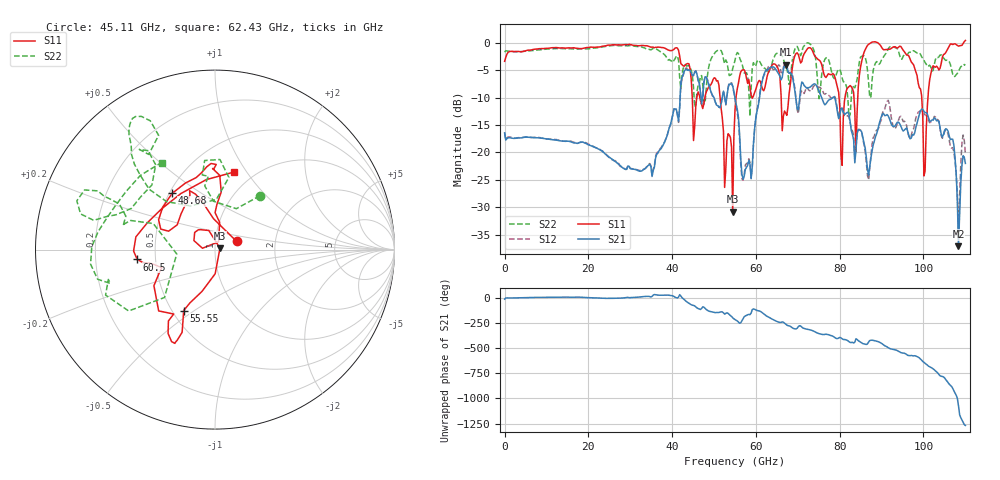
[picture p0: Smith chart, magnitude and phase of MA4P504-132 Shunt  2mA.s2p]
!Keysight Technologies,N5247B,US61255204,A.15.70.20
!Date: Friday, October 21, 2022 14:56:18
!Correction: S11(C  4-Port  )
!S31(C  4-Port  )
!S13(C  4-Port  )
!S33(C  4-Port  )
!S2P File: Measurements: S11, S31, S13, S33:
# Hz S  dB  R 50
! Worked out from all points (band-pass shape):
!   401 points, 10 MHz to 110 GHz, reference 50 ohm
!   highest |S21| = -3.99 dB at 67.1 GHz (marker M1); lowest = -37.1 dB at 108.4 GHz (marker M2)
!   |S21| within 3 dB of the highest: 42.15 GHz to 46.28 GHz (4.135 GHz wide, 9.35 % of centre); 61.5 GHz to 68.91 GHz (7.411 GHz wide, 11.4 % of centre)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
!   lowest |S11| = -30.8 dB at 54.46 GHz (marker M3), VSWR 1.06, Z = 52.8 + j0.811 ohm
!   |S11| at or under -10 dB: 51.45 GHz to 55.25 GHz (3.792 GHz wide, 7.11 % of centre); 66.02 GHz to 67.84 GHz (1.818 GHz wide, 2.72 % of centre); 79.85 GHz to 81.26 GHz (1.412 GHz wide, 1.75 % of centre)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
!   |S22| runs from -13.5 to 0.0 dB; largest |S21 - S12| = 0.24
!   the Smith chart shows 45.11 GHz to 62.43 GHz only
!   S11 on the Smith chart (normalised r, x): 45.11 GHz: 1.27, +0.12; 48.68 GHz: 0.52, +0.38; 55.55 GHz: 0.57, -0.45; 60.5 GHz: 0.39, -0.05; 62.43 GHz: 0.81, +0.88
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1e7  -3.37 -178.2  -16.43 -9.8  -16.39 -9.7  -1.68 -178.3
1.843332e10  -1.04 117.9  -18.11 8.6  -18.13 8.8  -1.08 124.4
3.685665e10  -0.77 115.2  -19.72 29.4  -19.58 29.3  -1.41 122.0
4.345605e10  -3.83 23.6  -4.88 -35.3  -4.58 -32.2  -4.23 83.0
4.51059e10  -17.82 21.0  -5.93 -72.1  -5.97 -71.1  -8.15 50.1
4.868058e10  -8.09 127.3  -7.44 -127.4  -7.28 -126.0  -4.62 135.2
5.445505e10  -30.84 15.5  -7.86 164.7  -7.94 163.8  -4.66 160.6
5.5005e10  -12.24 -107.4  -10.10 146.5  -10.34 144.7  -3.16 166.4
5.555495e10  -8.35 -117.2  -12.14 132.9  -12.74 132.2  -1.76 160.6
5.72048e10  -4.93 -115.3  -24.34 174.7  -23.99 -175.1  -5.50 159.4
6.05045e10  -7.20 -172.8  -11.67 -125.6  -11.31 -120.8  -3.12 -173.4
6.242932e10  -7.04 76.3  -4.99 -174.7  -5.21 -168.4  -4.89 121.6
6.71039e10  -12.80 -41.7  -3.99 101.3  -3.67 101.7  -4.35 45.6
7.342832e10  -1.33 138.6  -7.73 37.6  -8.44 35.9  -0.68 108.4
8.112762e10  -10.63 -29.4  -13.08 -52.3  -13.38 -53.1  -7.18 -125.0
8.525225e10  -3.34 38.5  -16.26 -86.7  -16.34 -85.4  -2.45 -23.6
9.185165e10  -1.16 90.7  -13.82 -139.8  -11.16 -134.0  -0.78 83.7
9.872602e10  -7.33 151.3  -13.87 131.7  -12.68 131.2  -1.77 177.1
1.003759e11  -23.40 -38.7  -12.71 70.3  -13.14 72.1  -3.58 -155.6
1.036756e11  -4.93 -33.9  -14.36 -40.3  -14.27 -37.4  -2.55 -90.0
1.083502e11  -0.59 22.4  -37.12 8.7  -34.42 13.2  -5.17 -5.1
1.1e11  0.45 54.4  -22.01 171.1  -20.19 173.0  -4.09 16.6
